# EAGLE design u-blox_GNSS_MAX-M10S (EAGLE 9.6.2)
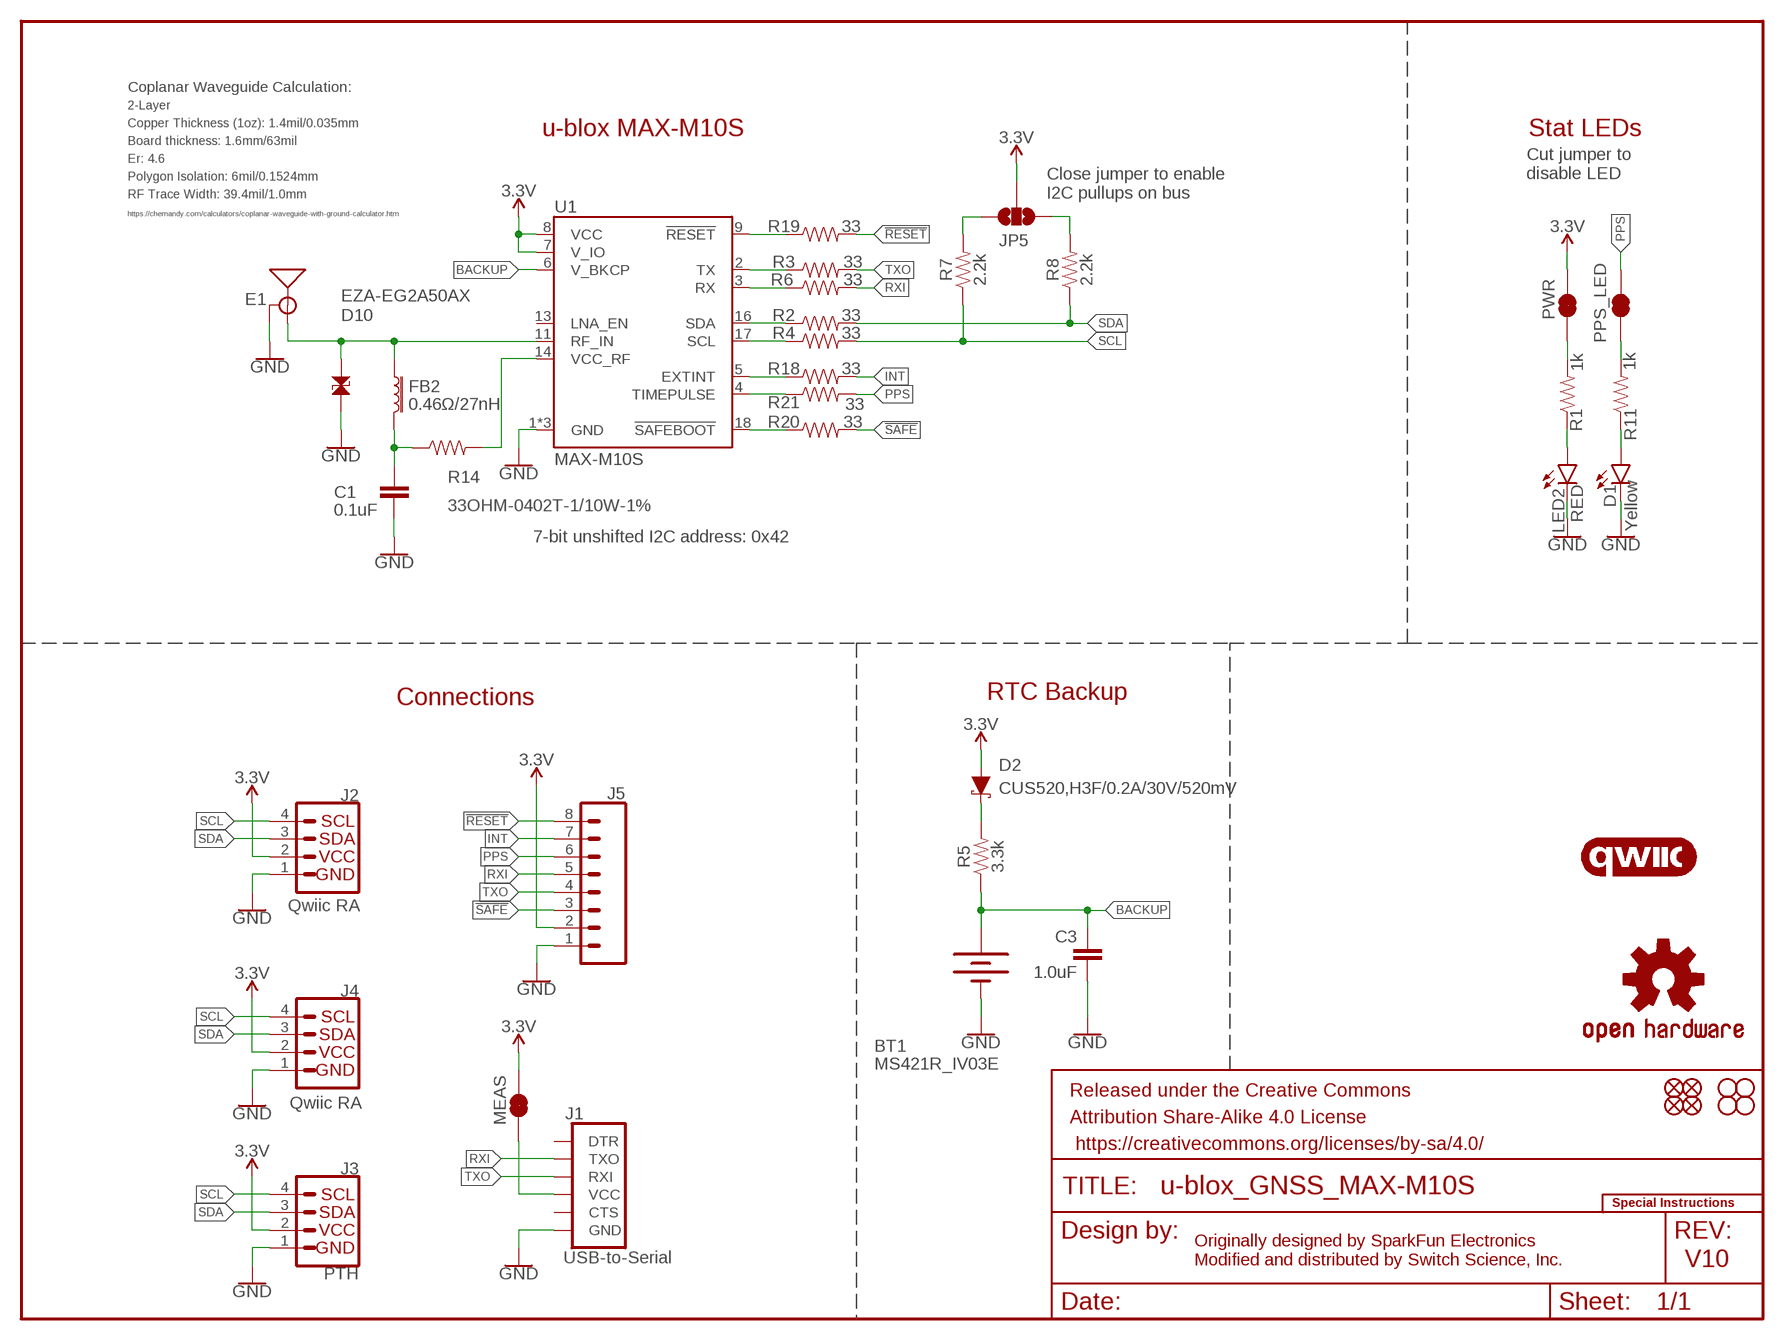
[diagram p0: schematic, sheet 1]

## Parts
BT1  MS421R_IV03E  RELOWABLE_BATTERY_MS421R  [MS421R_IV03E]
C1  0.1uF  47PF-0402_TIGHT-25V-5%-X7R  [0402-TIGHT]
C3  1.0uF  1.0UF-0603-16V-10%-X7R  [0603]
D1  Yellow  LED-YELLOW0603  [LED-0603]
D2  CUS520,H3F/0.2A/30V/520mV  DIODE-SCHOTTKY-PMEG4005EJ  [SOD-323]
D10  EZA-EG2A50AX  PESD0402-0402T  [0402-TIGHT]
E1  ANTENNA-SMA-GROUNDEDEDGE_SMA  [SMA-EDGE]
FB2  0.46Ω/27nH  FERRITE_BEAD-0402-2.66Ω-1GHZ  [0402-TIGHT]
FD1  FIDUCIALUFIDUCIAL  [FIDUCIAL-MICRO]
FD2  FIDUCIALUFIDUCIAL  [FIDUCIAL-MICRO]
FD3  FIDUCIALUFIDUCIAL  [FIDUCIAL-MICRO]
FD4  FIDUCIALUFIDUCIAL  [FIDUCIAL-MICRO]
FRAME1  FRAME-LETTER  [CREATIVE_COMMONS]
H1  STAND-OFF  [STAND-OFF]
H2  STAND-OFF  [STAND-OFF]
H3  STAND-OFF  [STAND-OFF]
H4  STAND-OFF  [STAND-OFF]
J1  USB-to-Serial  6_PIN_SERIAL_TARGET_NO_SILK  [1X06_NO_SILK]
J2  Qwiic RA  I2C_STANDARDQWIIC  [JST04_1MM_RA]
J3  PTH  I2C_STANDARD_NO_SILK  [1X04_NO_SILK]
J4  Qwiic RA  I2C_STANDARDQWIIC  [JST04_1MM_RA]
J5  CONN_08NO_SILK_DNP  [1X08_NO_SILK]
JP5  JUMPER-SMT_3_NO_SILK  [SMT-JUMPER_3_NO_SILK]
LED2  RED  LED-RED0603  [LED-0603]
LOGO1  OSHW-LOGOMINI  [OSHW-LOGO-MINI]
LOGO3  QWIIC_LOGO_5MM  [QWIIC_5MM]
MEAS  JUMPER-COMBO_2_NC_TRACE  [COMBO-JUMPER_2_NC_TRACE]
PPS_LED  JUMPER-SMT_2_NC_TRACE_SILK  [SMT-JUMPER_2_NC_TRACE_SILK]
PWR  JUMPER-SMT_2_NC_TRACE_SILK  [SMT-JUMPER_2_NC_TRACE_SILK]
R1  1k  1KOHM-0603-1/10W-1%  [0603]
R2  33  33OHM-0603-1/10W-1%  [0603]
R3  33  33OHM-0603-1/10W-1%  [0603]
R4  33  33OHM-0603-1/10W-1%  [0603]
R5  3.3k  3.3KOHM-0603-1/10W-1%  [0603]
R6  33  33OHM-0603-1/10W-1%  [0603]
R7  2.2k  2.2KOHM-0603-1/10W-1%  [0603]
R8  2.2k  2.2KOHM-0603-1/10W-1%  [0603]
R11  1k  1KOHM-0603-1/10W-1%  [0603]
R14  33OHM-0402T-1/10W-1%  [0402-TIGHT]
R18  33  33OHM-0603-1/10W-1%  [0603]
R19  33  33OHM-0603-1/10W-1%  [0603]
R20  33  33OHM-0603-1/10W-1%  [0603]
R21  33  33OHM-0603-1/10W-1%  [0603]
U1  MAX-M10S  [MAX-M10S]
U$2  SPECIAL_INSTRUCTIONS-ORDERING  [ORDERING_INSTRUCTIONS]

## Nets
3.3V [3.3V]: D2.A J2.2 J3.2(VCC) J4.2 J5.2 JP5.2 MEAS.2 MEAS.4 PWR.2 U1.7(V_IO) U1.8(VCC)
!RESET: J5.8 R19.2
!SAFE: J5.3 R20.2
ANT_VCC: C1.1 FB2.2 R14.1
BACKUP: BT1.+ C3.1 R5.1 U1.6(V_BKCP)
EXTINT_LV: R18.1 U1.5(EXTINT)
GND: BT1.- C1.2 C3.2 D1.C D10.2 E1.GND@0(GND) E1.GND@1(GND) E1.GND@2(GND) E1.GND@3(GND) J1.6(GND) J2.1 J3.1(GND) J4.1 J5.1 LED2.C U1.1(GND) U1.10(GND) U1.12(GND)
GPS_RF [RF]: D10.1 E1.SIG(SIGNAL) FB2.1 U1.11(RF_IN)
INT: J5.7 R18.2
N$1 [3.3V]: J1.4(VCC) MEAS.1 MEAS.3
N$2: D1.A R11.1
N$4: PPS_LED.1 R11.2
N$5: JP5.1 R8.2
N$6: D2.C R5.2
N$8: JP5.3 R7.2
N$10: LED2.A R1.1
N$17: PWR.1 R1.2
PPS: J5.6 PPS_LED.2 R21.2
PPS_LV: R21.1 U1.4(TIMEPULSE)
RST_LV: R19.1 U1.9(!RESET!)
RXI: J1.3(TXO) J5.5 R6.2
RXLV: R6.1 U1.3(RX)
SAFE_LV: R20.1 U1.18(!SAFEBOOT!)
SCL: J2.4 J3.4(SCL) J4.4 R4.2 R7.1
SCL_LV: R4.1 U1.17(SCL)
SDA: J2.3 J3.3(SDA) J4.3 R2.2 R8.1
SDA_LV: R2.1 U1.16(SDA)
TXLV: R3.1 U1.2(TX)
TXO: J1.2(RXI) J5.4 R3.2
VCC_RF: R14.2 U1.14(VCC_RF)
Unconnected: J1.1(DTR) J1.5(CTS) U1.13(LNA_EN)

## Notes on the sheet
- Coplanar Waveguide Calculation:
- 2-Layer
- Copper Thickness (1oz): 1.4mil/0.035mm | u-blox MAX-M10S | Stat LEDs
- Board thickness: 1.6mm/63mil
- Er: 4.6
- Cut jumper to 
  disable LED
- Polygon Isolation: 6mil/0.1524mm
- RF Trace Width: 39.4mil/1.0mm
- Close jumper to enable
  I2C pullups on bus
- https://chemandy.com/calculators/coplanar-waveguide-with-ground-calculator.htm
- 7-bit unshifted I2C address: 0x42
- Connections | RTC Backup
- Originally designed by SparkFun Electronics
  Modified and distributed by Switch Science, Inc.
- V10

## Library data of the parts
BT1 = SparkFun-Batteries:RELOWABLE_BATTERY: SEIKO Reflowable Lithium Batteries; PROD_ID: BAT-16685
C1 = SparkFun-Capacitors:47PF: 47pF ceramic capacitors; PROD_ID: CAP-15063; VALUE: 47pF
C3 = SparkFun-Capacitors:1.0UF: 1µF ceramic capacitors; PROD_ID: CAP-13930
D1 = SparkFun-LED:LED-YELLOW: Yellow SMD LED; PROD_ID: DIO-09003
D2 = SparkFun-DiscreteSemi:DIODE-SCHOTTKY: Schottky diode; PROD_ID: DIO-10955; VALUE: 0.5A/40V/420mV
D10 = SparkFun-DiscreteSemi:PESD0402: ESD protection diode; PROD_ID: DIO-15359
E1 = SparkFun-RF:ANTENNA-SMA-GROUNDED: SMA Antenna Connector w/ Ground; PROD_ID: CONN-08289
FB2 = SparkFun-Coils:FERRITE_BEAD: Ferrite Bead (blocks, cores, rings, chokes, etc.); PROD_ID: NDUC-15072; VALUE: 2.66Ω
FD1-FD4 = SparkFun-Aesthetics:FIDUCIAL: Fiducial Alignment Points
FRAME1 = SparkFun-Aesthetics:FRAME-LETTER: Schematic Frame - Letter
H1-H4 = SparkFun-Hardware:STAND-OFF: Stand Off
J1 = SparkFun-Connectors:6_PIN_SERIAL_TARGET: 6-pin header connection for use with the "FTDI BASIC" pinout - TARGET SIDE. Also known as "Arduino Serial Program Header". It is used to mate with our FTDI Basic serial programmers using the Arduino IDE. Note, this device has "TARGET" in the name. It is intended to be used on a design that contains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
J2 J4 = SparkFun-Connectors:I2C_STANDARD: SparkFun I2C Standard Pinout Header SparkFun has standardized on a pinout for all I2C based sensor breakouts. This pinout allows I2C boards to be plugged directly into the headers on Arduino Uno compatible boards, and to be daisy chained easily. Example SparkFun Products: SparkFun Atmospheric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; PROD_ID: CONN-13694; VALUE: Qwiic Right Angle
J3 = SparkX:I2C_STANDARD: SparkFun I2C Standard Pinout Header SparkFun has standardized on a pinout for all I2C based sensor breakouts. This pinout allows I2C boards to be plugged directly into the headers on Arduino Uno compatible boards, and to be daisy chained easily. Example SparkFun Products: SparkFun Atmospheric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
J5 = SparkFun-Connectors:CONN_08: Multi connection point. Often used as Generic Header-pin footprint for 0.1 inch spaced/style header connections On any of the 0.1 inch spaced packages, you can populate with these: Break Away Headers - Straight (PRT-00116) Break Away Male Headers - Right Angle (PRT-00553) Female Headers (PRT-00115)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
JP5 = SparkFun-Jumpers:JUMPER-SMT_3_NO: Normally open jumper This jumper has three pads in close proximity to each other. Apply solder to close the connection(s).
LED2 = SparkFun-LED:LED-RED: Red SMD LED; PROD_ID: DIO-00819
LOGO1 = SparkFun-Aesthetics:OSHW-LOGO: Open-Source Hardware (OSHW) Logo
LOGO3 = SparkFun-Aesthetics:QWIIC_LOGO: Qwiic Logos for placement on schematic and PCB. The 5.5mm silk logo is best for placing next to Qwiic connector.
MEAS = SparkFun-Jumpers:JUMPER-COMBO_2_NC_TRACE
PPS_LED PWR = SparkFun-Jumpers:JUMPER-SMT_2_NC_TRACE: Normally closed trace jumper
R1 R11 = SparkFun-Resistors:1KOHM: 1kΩ resistor; PROD_ID: RES-07856
R2-R4 R6 R18-R21 = SparkFun-Resistors:33OHM: 33Ω resistor; PROD_ID: RES-08270
R5 = SparkFun-Resistors:3.3KOHM: 3.3kΩ resistor; PROD_ID: RES-07851
R7 R8 = SparkFun-Resistors:2.2KOHM: 2.2kΩ resistor; PROD_ID: RES-08272
R14 = SparkFun-Resistors:33OHM: 33Ω resistor; PROD_ID: RES-14883
U1 = GNSS-MAX:MAX-M10S; PROD_ID: IC-15926
U$2 = SparkFun-Aesthetics:SPECIAL_INSTRUCTIONS: Special Ordering/Production Instructions Alert

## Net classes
2 3.3V: width 0.508 mm, drill 0.305 mm
3 RF: width 0.889 mm, drill 0.305 mm, clearance 0.203 mm

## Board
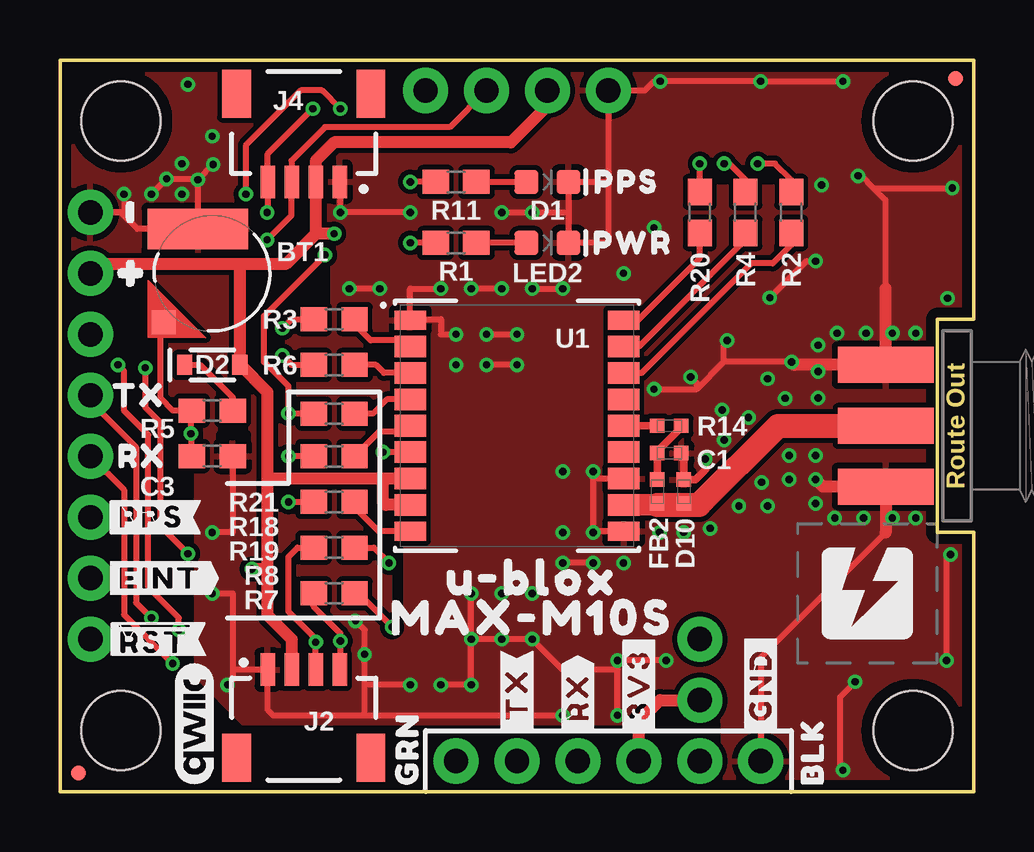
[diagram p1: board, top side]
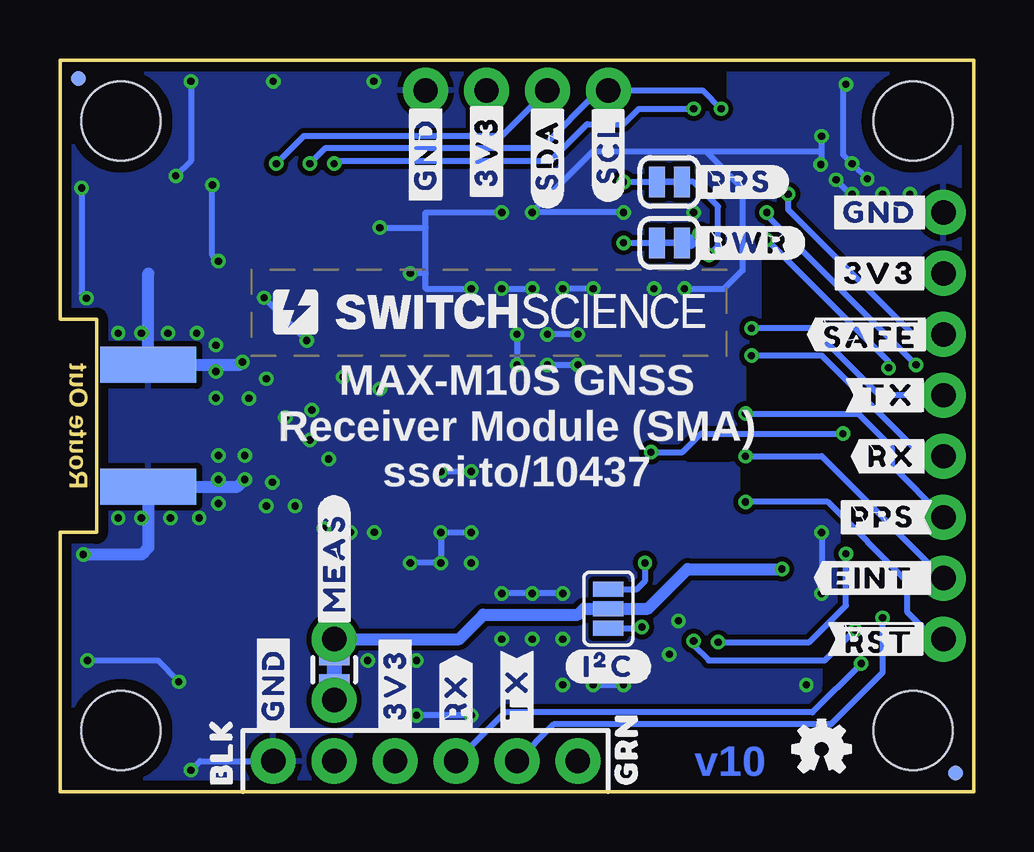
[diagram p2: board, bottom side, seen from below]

Size 38.1 x 30.48 mm. Coordinates in mm from the lower left corner, seen from the top.
Outline: 38.1,0 0,0 0,30.48 38.1,30.48 38.1,19.68 36.58,19.68 36.58,10.79 38.1,10.79 38.1,0
Copper layers (1*16): Top/Horz 0.035mm / dielectric 1.6mm / Bottom/Vert 0.035mm
Design rules "jlcpcb-2layers改": minimum track width 5mil, minimum drill 0.3mm, track to track 5mil, track to pad 5mil, pad to pad 5mil, via to via 5mil, smd to smd 5mil, copper to edge 0.4mm, drill to drill 6mil, minimum pad ring 10mil, minimum via ring 3mil, stop-mask expansion 2mil, vias tented up to drill 0.3mm, thermal gap 10mil
tKeepout: area 15.4,10.2 to 22.7,20.3
bKeepout: area 15.4,10.2 to 22.7,20.3
tRestrict: 11 lines
bRestrict: 10 lines

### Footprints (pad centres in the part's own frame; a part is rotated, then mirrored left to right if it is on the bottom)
MS421R_IV03E = smd 1 x 1: + 2.022,2.032 | smd 4.2 x 1.7: - 0.6,-1.85
0402-TIGHT = smd 0.6 x 0.6: 1 -0.5,0; 2 0.5,0
0603 = smd 1.1 x 1: 1 -0.85,0; 2 0.85,0
LED-0603 = smd 1 x 1: A -0.877,0; C 0.877,0
SOD-323 = smd 0.63 x 0.83: A 1.15,0; C -1.15,0
SMA-EDGE = smd 1.5 x 4: GND@0 -2.54,0; GND@1 2.54,0; SIG 0,0 | smd 1.5 x 4 bottom: GND@2 -2.54,0; GND@3 2.54,0
FIDUCIAL-MICRO = smd 0.635 x 0.635: 1 0,0
STAND-OFF = hole 3.302: 0,0
1X06_NO_SILK = drill 1.016 pad 1.88: 1 0,0; 2 2.54,0; 3 5.08,0; 4 7.62,0; 5 10.16,0; 6 12.7,0
JST04_1MM_RA = smd 0.6 x 1.35: 1 -1.5,0; 2 -0.5,0; 3 0.5,0; 4 1.5,0 | smd 1.2 x 2: NC1 2.8,-3.675; NC2 -2.8,-3.675
1X04_NO_SILK = drill 1.016 pad 1.88: 1 0,0; 2 2.54,0; 3 5.08,0; 4 7.62,0
1X08_NO_SILK = drill 1.016 pad 1.88: 1 0,0; 2 2.54,0; 3 5.08,0; 4 7.62,0; 5 10.16,0; 6 12.7,0; 7 15.24,0; 8 17.78,0
SMT-JUMPER_3_NO_SILK = smd 0.635 x 1.27: 1 -0.813,0; 2 0,0; 3 0.813,0
COMBO-JUMPER_2_NC_TRACE = smd 0.635 x 1.27: 1 -0.508,0; 2 0.508,0 | drill 1.016 pad 1.88: 3 -1.27,0; 4 1.27,0
SMT-JUMPER_2_NC_TRACE_SILK = smd 0.66 x 1.27: 1 -0.521,0; 2 0.521,0
MAX-M10S = smd 1.3 x 0.8: 1 4.45,-4.4; 9 4.45,4.4; 10 -4.45,4.4; 18 -4.45,-4.4 | smd 1.3 x 0.9: 2 4.45,-3.3; 3 4.45,-2.2; 4 4.45,-1.1; 5 4.45,0; 6 4.45,1.1; 7 4.45,2.2; 8 4.45,3.3; 11 -4.45,3.3; 12 -4.45,2.2; 13 -4.45,1.1; 14 -4.45,0; 15 -4.45,-1.1; 16 -4.45,-2.2; 17 -4.45,-3.3

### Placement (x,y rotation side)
BT1  6.35,21.59 180 top
C1  25.4,14.1 0 top
C3  6.35,13.97 0 top
D1  20.32,25.4 0 top
D2  6.35,17.78 0 top
D10  26,12.5 90 top
E1  34.42,15.24 270 top
FB2  24.9,12.5 90 top
FD1  0.76,0.76 0 top
FD2  0.76,0.76 0 bottom
FD3  37.34,29.72 0 top
FD4  37.34,29.72 0 bottom
FRAME1  not placed on the board
H1  35.56,2.54 0 top
H2  2.54,2.54 0 top
H3  2.54,27.94 0 top
H4  35.56,27.94 0 top
J1  16.51,1.27 0 top
J2  10.16,5.08 0 top
J3  22.86,29.21 180 top
J4  10.16,25.4 180 top
J5  1.27,24.13 270 top
JP5  15.24,7.62 270 bottom
LED2  20.32,22.86 0 top
LOGO1  6.35,1.78 0 bottom
LOGO3  5.59,2.79 90 top
MEAS  26.67,5.08 90 bottom
PPS_LED  12.7,25.4 0 bottom
PWR  12.7,22.86 0 bottom
R1  16.51,22.86 180 top
R2  30.48,24.13 90 top
R3  11.43,19.68 180 top
R4  28.57,24.13 90 top
R5  6.35,15.88 0 top
R6  11.43,17.78 180 top
R7  11.43,8.26 0 top
R8  11.43,10.16 0 top
R11  16.51,25.4 180 top
R14  25.4,15.24 180 top
R18  11.43,13.97 180 top
R19  11.43,12.06 180 top
R20  26.67,24.13 90 top
R21  11.43,15.75 180 top
U1  19.05,15.24 180 top
U$1  [#3V3#4]  24.13,4.45 90 top
U$2  not placed on the board
U$3  [#GND#5]  29.21,4.45 90 top
U$4  [BLK0]  31.37,1.65 90 top
U$5  [GRN1]  14.48,1.78 90 top
U$6  [PPS7]  23.62,25.4 0 top
U$7  [PWR6]  23.88,22.86 0 top
U$8  [#RX#2]  21.59,3.94 90 top
U$9  [#TX#3]  19.05,4.06 90 top
U$10  [#3V3#4]  3.94,21.59 0 bottom
U$11  [#GND#5]  3.94,24.13 0 bottom
U$12  [##RST##2]  3.94,6.35 0 bottom
U$13  [##SAFE##0]  4.32,19.05 0 bottom
U$14  [#PPS#1]  3.81,11.43 0 bottom
U$15  [#RX#1]  3.43,13.97 0 bottom
U$16  [#TX#0]  3.56,16.51 0 bottom
U$17  [LOGO_150MIL]  31.75,6.35 0 top
U$18  [MAX#M10S1]  19.68,7.24 0 top
U$19  [#0]  3.05,21.59 0 top
U$20  [U#BLOX0]  19.68,8.89 0 top
U$22  [#TX#3]  19.05,4.06 90 bottom
U$25  [#RX#2]  21.59,3.94 90 bottom
U$26  [#3V3#4]  24.13,4.45 90 bottom
U$27  [#GND#5]  29.21,4.45 90 bottom
U$28  [BLK0]  31.37,1.65 90 bottom
U$29  [GRN1]  14.48,1.78 90 bottom
U$30  [#I�C#0]  15.24,5.21 0 bottom
U$31  [#3V3#4]  20.32,26.67 90 bottom
U$32  [#SCL#1]  15.24,26.67 90 bottom
U$33  [#SDA#0]  17.78,26.54 90 bottom
U$34  [#GND#5]  22.86,26.54 90 bottom
U$35  [#PPS#0]  9.78,25.4 0 bottom
U$36  [#PWR#0]  9.4,22.86 0 bottom
U$39  [##RST##0]  3.94,6.35 0 top
U$40  [#1]  2.92,24.26 90 top
U$41  [#MEAS#0]  26.67,9.53 90 bottom
U$42  [#EINT#0]  4.19,8.89 0 top
U$43  [#PPS#1]  3.81,11.43 0 top
U$44  [RX2]  3.43,13.97 0 top
U$45  [TX3]  3.3,16.51 0 top
U$46  [#EINT_#0]  4.06,8.89 0 bottom
U$47  [LOGO_WITH_SSCI_18MM]  29.21,19.05 0 bottom

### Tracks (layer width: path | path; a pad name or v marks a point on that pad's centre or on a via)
3.3V  (via drill 0.3 pad 0.6)
  Top/Horz 0.508: J3.2 20.32,28.57 18.8,27.05 11.43,27.05 10.66,26.28 J4.2 10.66,23.23 | v11.43,23.24 v11.42,23.23 10.66,23.23 | 10.66,23.23 9.4,21.97 7.49,21.97 | J5.2 1.65,21.97 7.49,21.97 | 7.49,21.97 7.5,21.96 D2.A 8.64,16.64 8.64,12.95 | J2.2 9.66,6.34 8.64,7.37 8.64,9.4 | 8.64,12.95 8.64,9.4 | 8.64,9.4 8.51,9.27 v8,9.27 | U1.7 13.46,13.04 | 13.46,13.04 8.72,13.04 8.64,12.95 | U1.8 13.59,11.94 13.46,12.06 13.46,13.04
  Bottom/Vert 0.508: MEAS.2 MEAS.4 21.46,6.35 20.45,7.37 16.51,7.37 16.26,7.62 JP5.2 13.59,7.62 11.94,9.27 v8,9.27 | PWR.2 11.81,22.86 v11.43,23.24
!RESET  (via drill 0.3 pad 0.6)
  Top/Horz 0.254: v9.53,12.06 R19.2
  Bottom/Vert 0.254: J5.8 1.65,6.35 2.79,7.49 2.79,8.76 6.1,12.06 v9.53,12.06
!SAFE  (via drill 0.3 pad 0.6)
  Top/Horz 0.254: R20.2 v26.67,26.16 | v11.68,28.45 10.92,29.21 10.03,29.21 7.75,26.92 v7.75,24.89
  Bottom/Vert 0.254: v26.67,26.16 26.54,26.29 17.65,26.29 16.13,27.81 14.61,27.81 13.97,28.45 v11.68,28.45 | v7.75,24.89 7.75,24.26 2.54,19.05 J5.3
ANT_VCC
  Top/Horz 0.305: C1.1 | C1.1 FB2.2 | FB2.2 | R14.1 25.9,15.17 24.9,14.17 C1.1
BACKUP  (via drill 0.3 pad 0.6)
  Top/Horz 0.254: R5.1 5.46,15.88 | 5.46,15.88 4.7,15.88 4.19,16.38 4.19,19.29 BT1.+ | U1.6 v13.46,14.14 | 5.46,15.88 v5.46,14.91 5.46,14.01 C3.1
  Bottom/Vert 0.254: v13.46,14.14 12.15,14.14 11.38,14.91 v5.46,14.91
EXTINT_LV
  Top/Horz 0.254: U1.5 14.35,14.99 13.3,14.99 R18.1
GND  (via drill 0.3 pad 0.6)
  Top/Horz 0.254: 21.2,24.13 D1.C 22.86,25.4 | 21.2,24.13 LED2.C 22.86,22.86 22.86,25.4 | 21.2,24.13 v19.68,24.13 v18.41,24.13 | 22.86,25.4 J3.1 24.38,29.21 24.77,29.59 v25.02,29.59 v29.21,29.59 v32.64,29.59 | J4.1 11.68,25.38 v11.68,24.13 v14.61,24.13 | C3.2 7.2,10.79 v6.35,10.79 | 34.42,10.79 29.21,5.59 J1.6 | BT1.- 5.71,23.6 5.61,23.5 | v33.15,4.57 32.51,3.94 32.51,1.02 v32.64,0.89 | v36.96,5.46 36.96,9.7 v37.13,9.87 | v33.27,25.65 33.4,25.65 33.91,25.15 | 33.91,25.15 v37.2,25.15 | 34.42,20.95 34.42,24.64 33.91,25.15 | v6.35,8.26 7.2,8.26 7.2,5.08 | U1.12 22.23,13.04 | 22.23,13.04 v22.23,10.79 22.27,10.84 U1.10 | 22.23,13.04 v22.23,13.34 | v16.51,19.05 15.88,19.05 15.88,19.68 14.64,19.68 U1.1 14.6,20.95 14.61,20.95 v15.88,20.95 | v17.78,19.05 v19.05,19.05 | v19.05,17.78 v17.78,17.78 | v13.34,20.95 v12.06,20.95 | v19.68,20.95 v20.95,20.95 | v18.41,20.95 v17.14,20.95 | v22.23,9.53 v20.95,9.53 | BT1.- 3.23,23.44 2.54,24.13 J5.1 2.67,24.13 v2.67,24.89 | BT1.- v5.75,25.49 | v6.38,26.13 v5.75,25.49 | v5.75,25.49 5.71,25.53 v4.45,25.53 v3.81,24.89 | v30.5,17.9 27.68,17.9 | v24.77,16.76 26.54,16.76 | 27.68,17.9 26.54,16.76 | 26.54,16.76 26.54,17.02 v26.29,17.27 | 27.68,17.9 27.68,18.66 v27.81,18.8 | v29.59,20.57 31.11,22.1 v31.5,22.1 | 12.7,3.17 8.89,3.17 8.66,3.4 J2.1 7.2,5.08 | 12.7,3.17 12.7,4.45 | 12.7,4.45 v12.7,5.71 12.7,6.73 v12.32,7.11 | 12.7,3.17 v20.95,3.17 | v25.27,5.46 v23.24,5.46 23.24,5.08 | v23.24,3.17 23.24,5.08 | v17.14,6.35 v18.41,6.35 v19.68,6.35 20.95,5.08 23.24,5.08 | v15.88,4.45 v17.14,4.45 v17.14,6.35 | v17.14,6.35 v17.14,8.26 | v14.61,4.45 12.7,4.45 | v6.99,4.45 7.2,4.66 7.2,5.08
  Top/Horz 0.305: C1.2 26,14 D10.2 26.48,13 26.9,13.41 v26.9,13.86
  Top/Horz 0.508: 34.42,10.79 E1.GND@3 31.8,12.7 v31.5,13 | v30.5,17.9 30.62,17.78 E1.GND@2 34.42,20.95
  Bottom/Vert 0.254: v20.95,20.95 22.86,20.95 22.86,21.59 | v19.68,20.95 v18.41,20.95 | 22.86,21.59 22.86,23.5 | 22.86,23.5 22.86,24.13 v19.68,24.13 | v14.61,24.13 v18.41,24.13 15.88,26.67 11.18,26.67 | 11.18,26.67 9.65,25.15 9.65,21.72 10.41,20.95 v12.06,20.95 | v32.64,0.89 32.26,1.27 J1.6 | v36.96,5.46 34.04,5.46 v33.15,4.57 | v32.64,29.59 32.64,26.29 v33.27,25.65 | v37.2,25.15 37.2,20.75 v37,20.55 | v24.77,23.5 22.86,23.5 | 22.86,21.59 v23.5,21.59 | v6.35,10.79 v6.35,8.26 | v22.23,13.34 v20.95,13.34 | v20.95,10.79 v22.23,10.79 v22.23,9.53 v23.5,9.53 | v16.51,19.05 v17.78,19.05 | v19.05,19.05 v19.05,17.78 | v17.78,17.78 v16.51,17.78 | v15.88,20.95 v17.14,20.95 | v6.38,26.13 6.35,26.16 6.35,26.67 | 6.35,26.67 v6.35,27.3 | v4.45,25.53 v5.08,26.16 5.46,26.54 5.46,29.34 v5.33,29.46 | v5.75,25.49 5.15,24.89 v5.08,24.89 | v27.81,18.8 v29.59,20.57 | v31.5,22.1 31.75,22.35 v31.75,25.27 | 11.18,26.67 6.35,26.67 | v20.95,3.17 v23.24,3.17 | v17.14,8.26 v18.41,8.26 v19.68,8.26 | v15.88,4.45 v14.61,4.45
  Bottom/Vert 0.508: v30.5,17.9 30.62,17.78 E1.GND@2 34.42,21.59 | v30.4,13 30.7,12.7 E1.GND@3 34.42,10.16 34.7,9.87 v37.13,9.87
  other vias: 25,10.8 26,10.8 29.5,11.9 27.6,15.9 28.3,11.9 32.3,11.4 31.5,12 31.6,16.4 29.5,17.2 31.5,14 31.6,17.5 30.4,14 28.7,15.58 30.23,16.38 33.5,11.4 34.7,11.4 35.67,11.4 32.4,19.1 33.6,19.1 34.7,19.1 35.67,19.1 31.6,18.6 27.69,14.65 27.11,10.96 29.25,12.88
  pour Top/Horz (isolate 0.203, rank 4): 0,0 0,30.48 38.1,30.48 38.1,0
  pour Bottom/Vert (isolate 0.203, rank 4): 0,0 0,30.48 38.1,30.48 38.1,0
GPS_RF
  Top/Horz 0.889: FB2.1 D10.1 26.06,11.94
  Top/Horz 0.9: U1.11 24.9,11.94
  Top/Horz 1: E1.SIG 29.94,15.24 26.64,11.94 26.06,11.94 24.9,11.94
INT  (via drill 0.3 pad 0.6)
  Top/Horz 0.254: R18.2 v9.53,13.97
  Bottom/Vert 0.254: v9.53,13.97 6.35,13.97 J5.7
N$1
  Top/Horz 0.508: J1.4 24.13,2.92 25.02,3.81 MEAS.3
  Bottom/Vert 0.508: MEAS.1 MEAS.3
N$2
  Top/Horz 0.254: R11.1 D1.A
N$4  (via drill 0.3 pad 0.6)
  Top/Horz 0.254: R11.2 v14.61,25.4
  Bottom/Vert 0.254: v14.61,25.4 PPS_LED.1
N$5  (via drill 0.3 pad 0.6)
  Top/Horz 0.254: R8.2 13.08,10.16 v13.72,9.53
  Bottom/Vert 0.254: v13.72,9.53 13.72,8.76 14.05,8.43 JP5.1
N$6
  Top/Horz 0.254: D2.C 5.84,17.78 7.2,16.42 R5.2
N$8  (via drill 0.3 pad 0.6)
  Top/Horz 0.254: v13.84,6.86 12.45,8.26 R7.2
  Bottom/Vert 0.254: JP5.3 13.89,6.81 v13.84,6.86
N$10
  Top/Horz 0.254: LED2.A R1.1
N$17  (via drill 0.3 pad 0.6)
  Top/Horz 0.254: R1.2 v14.61,22.86
  Bottom/Vert 0.254: v14.61,22.86 PWR.1
PPS  (via drill 0.3 pad 0.6)
  Top/Horz 0.254: R21.2 v9.53,15.75 9.53,16.89 8.51,17.91 8.51,19.81 v11.05,22.35
  Bottom/Vert 0.254: v9.53,15.75 4.83,15.75 3.43,14.35 3.43,13.59 J5.6 | v11.05,22.35 10.67,22.73 10.67,24.38 11.68,25.4 PPS_LED.2
PPS_LV
  Top/Horz 0.254: U1.4 13.63,16.34 13.04,15.75 R21.1
RST_LV
  Top/Horz 0.254: U1.9 13.29,10.84 12.28,11.85 R19.1
RXI  (via drill 0.3 pad 0.6)
  Top/Horz 0.254: v9.27,18.16 9.65,17.78 R6.2 | J5.5 2.67,12.57 2.67,7.37 v4.7,5.33
  Bottom/Vert 0.254: J5.5 2.16,13.97 6.35,18.16 v9.27,18.16 | v4.7,5.33 6.73,3.3 19.56,3.3 J1.3
RXLV
  Top/Horz 0.254: U1.3 13.51,17.44 13.17,17.78 R6.1
SAFE_LV
  Top/Horz 0.254: U1.18 24.09,19.64 26.67,22.23 R20.1
SCL  (via drill 0.3 pad 0.6)
  Top/Horz 0.254: v27.69,26.16 27.9,26.16 28.57,25.49 R4.2 | J2.4 11.69,5.11 v11.69,6.27 11.69,6.6 10.58,7.71 R7.1 | v4.95,6.73 4.95,7.24 3.68,8.51 3.68,14.86 2.67,15.88 2.67,17.53 v2.41,17.78 | v10.54,28.45 8.66,26.57 J4.4 8.66,24.15 v8.64,24.13
  Bottom/Vert 0.254: v27.69,26.16 27.05,26.8 18.03,26.8 15.62,29.21 J3.4 11.3,29.21 v10.54,28.45 | v11.69,6.27 11.69,6.1 11.05,5.46 6.22,5.46 v4.95,6.73 | v2.41,17.78 8.64,24 v8.64,24.13
SCL_LV
  Top/Horz 0.254: R4.1 28.57,22.99 24.13,18.54 U1.17
SDA  (via drill 0.3 pad 0.6)
  Top/Horz 0.254: R2.2 30.48,25.49 29.81,26.16 v29.08,26.16 | J2.3 v10.66,6.22 10.66,6.36 9.53,7.49 9.53,9.78 9.91,10.16 R8.1 | v3.56,17.65 3.56,16 4.19,15.37 4.19,11.05 v5.33,9.91 | J3.3 16.26,27.69 11.05,27.69 9.65,26.29 J4.3 | v8.64,22.99 9.65,24 J4.3 | J4.3
  Bottom/Vert 0.254: J3.3 19.68,27.3 27.94,27.3 v29.08,26.16 | v10.66,6.22 6.86,6.22 5.33,7.75 v5.33,9.91 | v3.56,17.65 3.56,17.91 v8.64,22.99
SDA_LV
  Top/Horz 0.254: U1.16 24.26,17.44 28.83,22.01 29.72,22.01 30.48,22.77 R2.1
TXLV
  Top/Horz 0.254: U1.2 14.35,18.79 12.96,18.79 12.28,19.47 R3.1
TXO  (via drill 0.3 pad 0.6)
  Top/Horz 0.254: v9.27,19.3 9.65,19.68 R3.2 | J5.4 1.27,16.26 3.17,14.35 3.17,7.87 v3.81,7.24
  Bottom/Vert 0.254: J5.4 3.94,16.51 6.73,19.3 v9.27,19.3 | v3.81,7.24 3.81,4.95 5.97,2.79 17.53,2.79 J1.2
VCC_RF
  Top/Horz 0.305: U1.14 R14.2

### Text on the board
Bottom/Vert: v10
bPlace: MAX-M10S GNSS / Receiver Module (SMA) / ssci.to/10437
Milling: Route Out
Measures: Measurements in inches
tDocu: Board thickness is 1.6mm | 2 Layer Board | N. Seidle | Originally designed by SparkFun Electronics / Modified and distributed by Switch Science, Inc.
